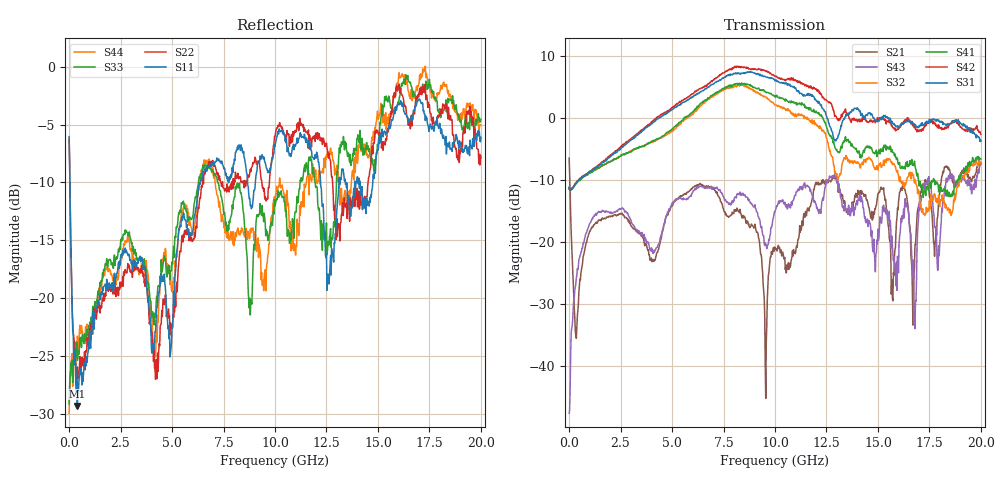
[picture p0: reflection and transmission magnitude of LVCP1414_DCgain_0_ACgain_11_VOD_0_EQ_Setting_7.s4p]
!Agilent Technologies,N5230A,MY46400459,A.07.50.48
!Agilent N5230A: A.07.50.48
!Date: Tuesday, April 17, 2012 18:43:29
!Correction: S11(Full 4 Port(1,2,3,4))
!S12(Full 4 Port(1,2,3,4))
!S13(Full 4 Port(1,2,3,4))
!S14(Full 4 Port(1,2,3,4))
!S21(Full 4 Port(1,2,3,4))
!S22(Full 4 Port(1,2,3,4))
!S23(Full 4 Port(1,2,3,4))
!S24(Full 4 Port(1,2,3,4))
!S31(Full 4 Port(1,2,3,4))
!S32(Full 4 Port(1,2,3,4))
!S33(Full 4 Port(1,2,3,4))
!S34(Full 4 Port(1,2,3,4))
!S41(Full 4 Port(1,2,3,4))
!S42(Full 4 Port(1,2,3,4))
!S43(Full 4 Port(1,2,3,4))
!S44(Full 4 Port(1,2,3,4))
!S4P File: Measurements: <S11,S12,S13,S14>,
!<S21,S22,S23,S24>,
!<S31,S32,S33,S34>,
!<S41,S42,S43,S44>:
# Hz S  dB  R 50
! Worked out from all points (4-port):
!   801 points, 300 kHz to 20 GHz, reference 50 ohm
!   strongest paths, dB at 300 kHz, 5 GHz, 10 GHz, 15 GHz, 20 GHz:
!     S31: -11.2, 1.3, 6.0, -0.6, -3.8
!     S42: -11.5, 1.7, 6.7, -0.1, -2.7
!     S41: -11.2, -1.8, 3.4, -5.5, -6.7
!     S32: -11.4, -2.2, 2.1, -8.4, -7.1
!     S43: -47.7, -13.8, -15.2, -17.9, -7.4
!     S21: -6.5, -14.1, -21.1, -12.2, -7.4
!   lowest |S11| = -29.3 dB at 400.3 MHz (marker M1), VSWR 1.07, Z = 53.2 + j1.59 ohm
!   |S11| at or under -10 dB: 37.86 MHz to 6.363 GHz (6.325 GHz wide, 198 % of centre); 12.21 GHz to 13.11 GHz (898.1 MHz wide, 7.09 % of centre); 14.13 GHz to 14.75 GHz (615 MHz wide, 4.26 % of centre)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
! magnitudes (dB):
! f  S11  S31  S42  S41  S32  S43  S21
! 300 kHz  -6.0  -11.2  -11.5  -11.2  -11.4  -47.7  -6.5
! 400.3 MHz  -29.3  -10.3  -10.2  -10.3  -10.3  -24.3  -32.0
! 10 GHz  -6.9  6.0  6.7  3.4  2.1  -15.2  -21.1
! 12.7 GHz  -16.3  -1.6  2.4  -2.8  -5.9  -9.6  -10.3
! 16.78 GHz  -3.8  -1.0  -1.6  -7.0  -10.5  -32.7  -24.2
! 17.33 GHz  -4.3  -0.7  -1.3  -12.5  -15.4  -10.7  -10.6
! 20 GHz  -6.1  -3.8  -2.7  -6.7  -7.1  -7.4  -7.4
